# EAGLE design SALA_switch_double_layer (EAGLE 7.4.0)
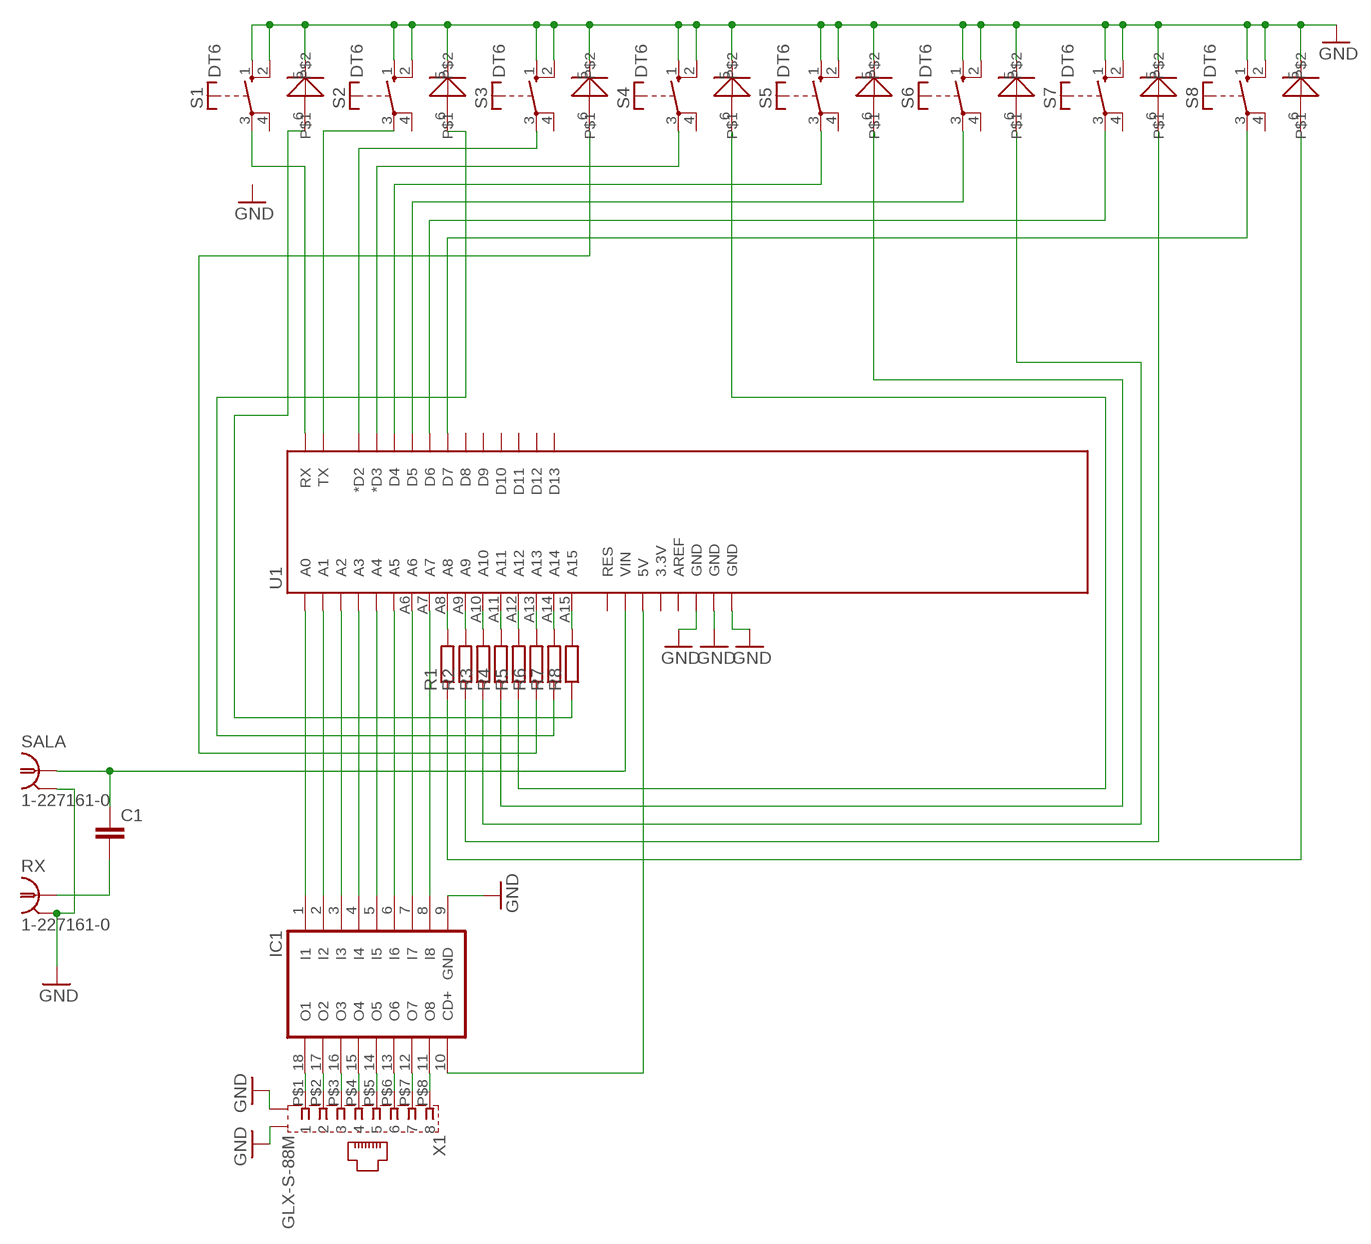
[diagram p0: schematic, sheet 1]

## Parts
C1  C-EU025-024X044  [C025-024X044]
IC1  ULN2803A  [DIL18]
R1  R-EU_R0805  [R0805]
R2  R-EU_R0805  [R0805]
R3  R-EU_R0805  [R0805]
R4  R-EU_R0805  [R0805]
R5  R-EU_R0805  [R0805]
R6  R-EU_R0805  [R0805]
R7  R-EU_R0805  [R0805]
R8  R-EU_R0805  [R0805]
RX  1-227161-0  [AMP_227161]
S1  DT6  [DT6]
S2  DT6  [DT6]
S3  DT6  [DT6]
S4  DT6  [DT6]
S5  DT6  [DT6]
S6  DT6  [DT6]
S7  DT6  [DT6]
S8  DT6  [DT6]
SALA  1-227161-0  [AMP_227161]
U1  ARDUINO_MEGA_SHIELD  [ARDUINO_MEGA_SHIELD]
X1  GLX-S-88M  [GLX-S-88M]

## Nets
GND: IC1.9(GND) RX.2 S1.1(S) S1.2(S) S1.5 S2.1(S) S2.2(S) S2.5 S3.1(S) S3.2(S) S3.5 S4.1(S) S4.2(S) S4.5 S5.1(S) S5.2(S) S5.5 S6.1(S) S6.2(S) S6.5 S7.1(S) S7.2(S) S7.5 S8.1(S) S8.2(S) S8.5 SALA.2 X1.P$9(S1) X1.P$10(S2)
GND@0: U1.GND@0(GND) ; supply symbol labelled GND
GND@1: U1.GND@1(GND) ; supply symbol labelled GND
GND@2: U1.GND@2(GND) ; supply symbol labelled GND
N$1: S1.3(P) U1.RX
N$2: S2.3(P) U1.TX
N$3: S3.3(P) U1.D2(*D2)
N$4: S4.3(P) U1.D3(*D3)
N$5: S5.3(P) U1.D4
N$6: S6.3(P) U1.D5
N$7: S7.3(P) U1.D6
N$8: S8.3(P) U1.D7
N$9: IC1.1(I1) U1.A0
N$10: IC1.2(I2) U1.A1
N$11: IC1.3(I3) U1.A2
N$12: IC1.4(I4) U1.A3
N$13: IC1.5(I5) U1.A4
N$14: IC1.6(I6) U1.A5
N$15: IC1.7(I7) U1.A6
N$16: IC1.8(I8) U1.A7
N$17: R1.2 U1.A8
N$18: R2.2 U1.A9
N$19: R3.2 U1.A10
N$20: R4.2 U1.A11
N$21: R5.2 U1.A12
N$22: R6.2 U1.A13
N$23: R7.2 U1.A14
N$24: R8.2 U1.A15
N$25: R8.1 S1.6
N$26: R7.1 S2.6
N$27: R5.1 S4.6
N$28: R6.1 S3.6
N$29: R3.1 S6.6
N$30: R2.1 S7.6
N$31: C1.1 SALA.1 U1.VIN
N$32: R1.1 S8.6
N$34: R4.1 S5.6
N$35: IC1.10(CD+) U1.5V@0(5V)
N$36: IC1.18(O1) X1.P$1
N$37: IC1.17(O2) X1.P$2
N$38: IC1.16(O3) X1.P$3
N$39: IC1.15(O4) X1.P$4
N$40: IC1.14(O5) X1.P$5
N$41: IC1.13(O6) X1.P$6
N$42: IC1.12(O7) X1.P$7
N$43: IC1.11(O8) X1.P$8
N$44: C1.2 RX.1
Unconnected: S1.4(P) S2.4(P) S3.4(P) S4.4(P) S5.4(P) S6.4(P) S7.4(P) S8.4(P) U1.3.3V U1.AREF U1.D8 U1.D9 U1.D10 U1.D11 U1.D12 U1.D13 U1.RES

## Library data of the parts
C1 = resistor:C-EU: CAPACITOR, European symbol
IC1 = uln-udn:ULN2803A: DRIVER ARRAY
R1-R8 = resistor:R-EU_: RESISTOR, European symbol
RX SALA = con-coax:?227161*: JACK, RIGHT ANGLE, 50 OHM, PCB, BNC; MF: TYCO ELECTRONICS; MPN: 1-227161; OC_FARNELL: unknown; OC_NEWARK: 33B3200
S1-S8 = switch-misc:DT: ITT SWITCH
U1 = RepRapjr:ARDUINO_MEGA_SHIELD
X1 = con-kycon:GLX-S-88M: Mod. Jack, Right Angle, 8 posiotion, 8 contatcs RJ45 Source: GLX-S-88M.pdf; OC_FARNELL: unknown; OC_NEWARK: unknown

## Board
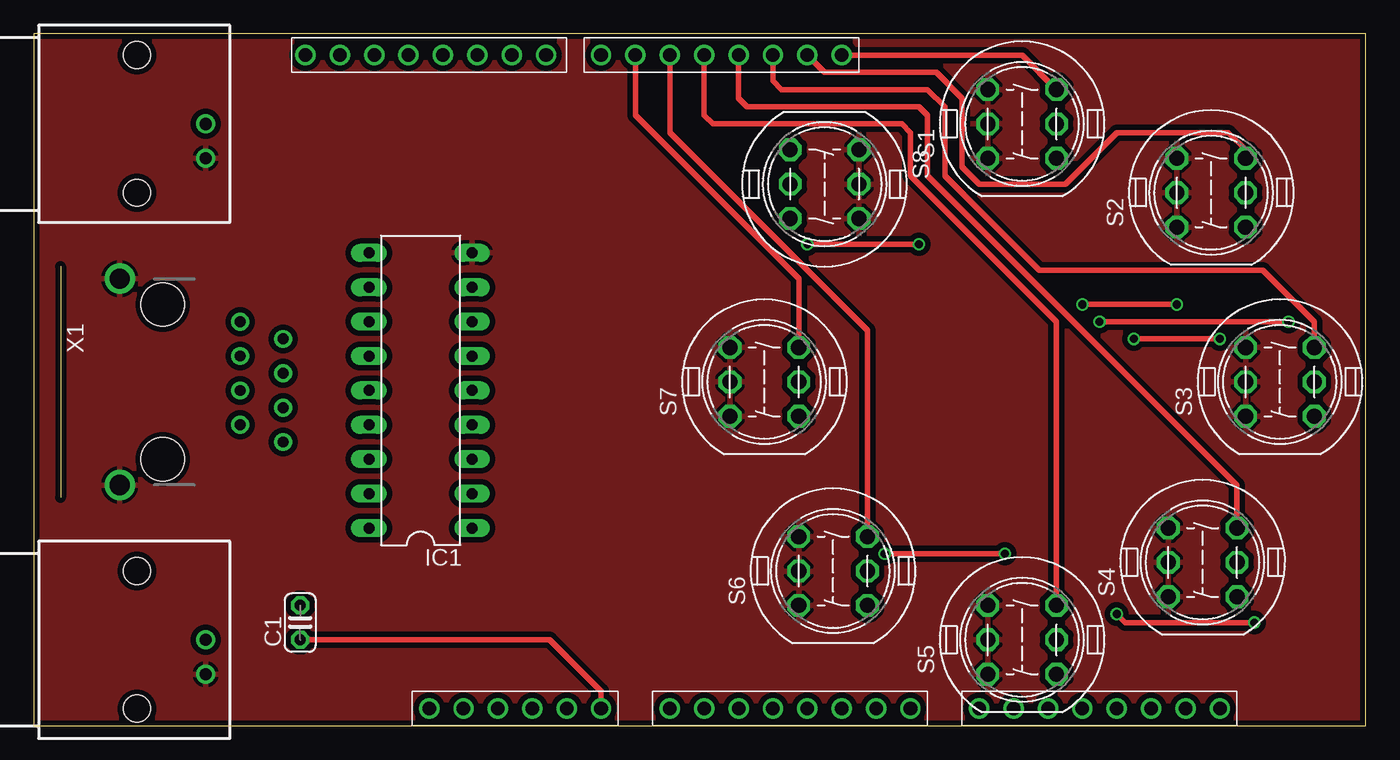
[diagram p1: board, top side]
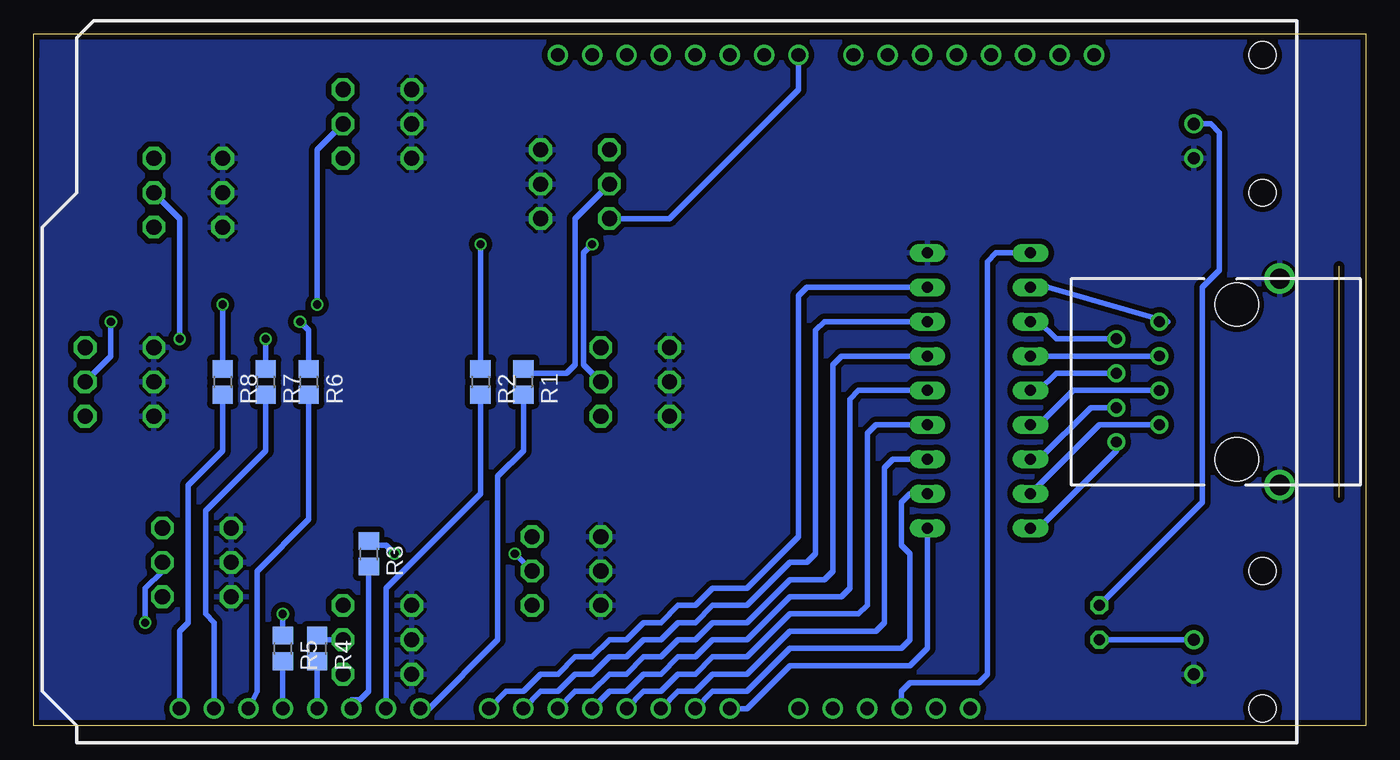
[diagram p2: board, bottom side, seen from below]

Size 98.41 x 51.1 mm. Coordinates in mm from the lower left corner, seen from the top.
Outline: 0,0 98.41,0 98.41,51.1 0,51.1 0,0
Copper layers (1*16): Top 0.035mm / dielectric 1.5mm / Bottom 0.035mm
Design rules "SeeedStudio_2layer_DRU_no_angle_20140221": minimum track width 6mil, minimum drill 12mil, track to track 6mil, track to pad 6mil, pad to pad 6mil, via to via 6mil, smd to smd 0mil, copper to edge 10mil, drill to drill 10mil, minimum pad ring 10mil, minimum via ring 6mil, stop-mask expansion 2mil, vias tented up to drill 100mil, thermal gap 10mil

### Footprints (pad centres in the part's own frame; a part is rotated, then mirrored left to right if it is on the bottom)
C025-024X044 = drill 0.813 octagon: 1 -1.27,0; 2 1.27,0
DIL18 = drill 0.813 long: 1 -10.16,-3.81; 2 -7.62,-3.81; 3 -5.08,-3.81; 4 -2.54,-3.81; 5 0,-3.81; 6 2.54,-3.81; 7 5.08,-3.81; 8 7.62,-3.81; 9 10.16,-3.81; 10 10.16,3.81; 11 7.62,3.81; 12 5.08,3.81; 13 2.54,3.81; 14 0,3.81; 15 -2.54,3.81; 16 -5.08,3.81; 17 -7.62,3.81; 18 -10.16,3.81
R0805 = smd 1.3 x 1.5: 1 -0.95,0; 2 0.95,0
AMP_227161 = drill 0.9 pad 1.27: 1 0,-5.08; 2 -2.54,-5.08 | hole 2: -5.08,0; 5.08,0
DT6 = drill 1.118 octagon: 1 -2.54,2.54; 2 2.54,2.54; 3 2.54,-2.54; 4 -2.54,-2.54; 5 0,2.54; 6 0,-2.54
ARDUINO_MEGA_SHIELD = drill 1 pad 1.422: 3.3V 50.8,26.67; 5V@0 50.8,29.21; A0 50.8,41.91; A1 50.8,44.45; A2 50.8,46.99; A3 50.8,49.53; A4 50.8,52.07; A5 50.8,54.61; A6 50.8,57.15; A7 50.8,59.69; A8 50.8,64.77; A9 50.8,67.31; A10 50.8,69.85; A11 50.8,72.39; A12 50.8,74.93; A13 50.8,77.47; A14 50.8,80.01; A15 50.8,82.55; AREF 2.54,14.986; D2 2.54,49.53; D3 2.54,46.99; D4 2.54,44.45; D5 2.54,41.91; D6 2.54,39.37; D7 2.54,36.83; D8 2.54,32.766; D9 2.54,30.226; D10 2.54,27.686; D11 2.54,25.146; D12 2.54,22.606; D13 2.54,20.066; GND@0 50.8,31.75; GND@1 50.8,34.29; GND@2 2.54,17.526; RES 50.8,24.13; RX 2.54,54.61; TX 2.54,52.07; VIN 50.8,36.83
GLX-S-88M = drill 0.8: P$1 4.445,3.175; P$2 3.175,0; P$3 1.905,3.175; P$4 0.635,0; P$5 -0.635,3.175; P$6 -1.905,0; P$7 -3.175,3.175; P$8 -4.445,0 | drill 1.5: P$9 -7.62,-8.89; P$10 7.62,-8.89 | hole 3.2: -5.715,-5.715; 5.715,-5.715

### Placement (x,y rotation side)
C1  19.69,7.62 90 top
IC1  28.58,24.76 90 top
R1  62.23,25.4 270 bottom
R2  65.41,25.4 270 bottom
R3  73.66,12.7 270 bottom
R4  77.47,5.71 270 bottom
R5  80.01,5.71 270 bottom
R6  78.11,25.4 270 bottom
R7  81.28,25.4 270 bottom
R8  84.45,25.4 270 bottom
RX  7.62,44.45 90 top
S1  73.03,44.45 90 top
S2  87,39.37 90 top
S3  92.08,25.4 90 top
S4  86.36,12.06 90 top
S5  73.03,6.35 90 top
S6  59.06,11.43 90 top
S7  53.98,25.4 90 top
S8  58.42,40.01 270 top
SALA  7.62,6.35 90 top
U1  5.08,52.07 270 top
X1  15.24,25.4 270 top

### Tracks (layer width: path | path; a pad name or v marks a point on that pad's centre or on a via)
GND
  pour Bottom (isolate 0.406): 0,50.8 97.79,50.8 98.42,-0.64 0,0
  pour Top (isolate 0.406): 0,50.8 98.42,50.8 98.42,-0.64 0,0
N$1
  Top 0.406: S1.3 73.03,49.53 U1.RX
N$2
  Top 0.406: S2.3 89.53,42.54 88.27,43.81 80.01,43.81 76.2,40.01 69.85,40.01 68.58,41.27 68.58,46.35 66.67,48.26 58.42,48.26 U1.TX
N$3
  Top 0.406: S3.3 94.61,29.84 90.81,33.65 74.3,33.65 67.31,40.64 67.31,45.72 66.04,46.99 55.25,46.99 54.61,47.62 U1.D2
N$4
  Top 0.406: S4.3 88.9,17.78 66.04,40.64 66.04,45.09 65.41,45.72 52.7,45.72 52.07,46.35 U1.D3
N$5
  Top 0.406: S5.3 75.56,29.84 64.77,40.64 64.77,43.81 64.14,44.45 50.17,44.45 49.53,45.09 U1.D4
N$6
  Top 0.406: S6.3 61.59,29.21 46.99,43.81 U1.D5
N$7
  Top 0.406: S7.3 56.52,33.02 44.45,45.09 U1.D6
N$8
  Bottom 0.406: S8.3 51.44,37.46 41.91,46.99 U1.D7
N$9
  Bottom 0.406: IC1.1 32.39,5.71 33.66,4.45 42.55,4.45 45.72,1.27 U1.A0
N$10
  Bottom 0.406: IC1.2 33.66,17.14 34.29,16.51 34.29,13.33 33.66,12.7 33.66,6.35 34.29,5.71 42.55,5.71 45.72,2.54 48.26,2.54 U1.A1
N$11
  Bottom 0.406: IC1.3 34.93,19.68 35.56,19.05 35.56,7.62 36.2,6.98 42.55,6.98 45.72,3.81 48.26,3.81 49.53,2.54 50.8,2.54 U1.A2
N$12
  Bottom 0.406: IC1.4 36.2,22.22 36.83,21.59 36.83,8.89 37.47,8.25 42.55,8.25 45.72,5.08 48.26,5.08 49.53,3.81 50.8,3.81 52.07,2.54 53.34,2.54 U1.A3
N$13
  Bottom 0.406: IC1.5 37.47,24.76 38.1,24.13 38.1,10.16 38.73,9.52 42.55,9.52 45.72,6.35 48.26,6.35 49.53,5.08 50.8,5.08 52.07,3.81 53.34,3.81 54.61,2.54 55.88,2.54 U1.A4
N$14
  Bottom 0.406: IC1.6 38.73,27.3 39.37,26.67 39.37,11.43 40.01,10.79 42.55,10.79 45.72,7.62 48.26,7.62 49.53,6.35 50.8,6.35 52.07,5.08 53.34,5.08 54.61,3.81 55.88,3.81 57.15,2.54 58.42,2.54 U1.A5
N$15
  Bottom 0.406: IC1.7 40.01,29.84 40.64,29.21 40.64,12.7 41.27,12.06 42.55,12.06 45.72,8.89 48.26,8.89 49.53,7.62 50.8,7.62 52.07,6.35 53.34,6.35 54.61,5.08 55.88,5.08 57.15,3.81 58.42,3.81 59.69,2.54 60.96,2.54 U1.A6
N$16
  Bottom 0.406: IC1.8 41.27,32.38 41.91,31.75 41.91,13.97 45.72,10.16 48.26,10.16 49.53,8.89 50.8,8.89 52.07,7.62 53.34,7.62 54.61,6.35 55.88,6.35 57.15,5.08 58.42,5.08 59.69,3.81 60.96,3.81 62.23,2.54 63.5,2.54 U1.A7
N$17
  Bottom 0.406: R1.2 62.23,20.32 64.14,18.41 64.14,6.35 69.22,1.27 U1.A8
N$18
  Bottom 0.406: R2.2 65.41,17.14 72.39,10.16 U1.A9
N$19
  Bottom 0.406: R3.2 73.66,2.54 74.3,1.9 74.93,1.9 U1.A10
N$20
  Bottom 0.406: U1.A11 R4.2
N$21
  Bottom 0.406: U1.A12 R5.2
N$22
  Bottom 0.406: R6.2 78.11,15.24 81.92,11.43 81.92,2.54 U1.A13
N$23
  Bottom 0.406: R7.2 81.28,20.32 85.73,15.88 85.73,8.25 85.09,7.62 U1.A14
N$24
  Bottom 0.406: R8.2 84.45,20.32 87,17.78 87,7.62 87.63,6.98 U1.A15
N$25  (via drill 0.6)
  Top 0.406: v84.45,31.12 v77.47,31.12
  Bottom 0.406: S1.6 77.47,42.54 v77.47,31.12 | R8.1 v84.45,31.12
N$26  (via drill 0.6)
  Top 0.406: v81.28,28.57 v87.63,28.57
  Bottom 0.406: S2.6 87.63,37.46 v87.63,28.57 | R7.1 v81.28,28.57
N$27  (via drill 0.6)
  Top 0.406: v90.17,7.62 80.64,7.62 v80.01,8.25
  Bottom 0.406: S4.6 88.9,11.43 90.17,10.16 v90.17,7.62 | R5.1 v80.01,8.25
N$28  (via drill 0.6)
  Top 0.406: v78.74,29.84 v92.71,29.84
  Bottom 0.406: S3.6 92.71,27.3 v92.71,29.84 | v78.74,29.84 78.11,29.21 R6.1
N$29  (via drill 0.6)
  Top 0.406: v71.75,12.7 v62.86,12.7
  Bottom 0.406: v62.86,12.7 S6.6 | v71.75,12.7 72.39,13.33 73.66,13.33 R3.1
N$30  (via drill 0.6)
  Top 0.406: v65.41,35.56 v57.15,35.56
  Bottom 0.406: S7.6 57.78,26.67 57.78,34.92 v57.15,35.56 | R2.1 v65.41,35.56
N$31
  Top 0.406: U1.VIN 41.91,2.54 38.1,6.35 C1.1
  Bottom 0.406: C1.1 SALA.1
N$32
  Bottom 0.406: S8.6 58.42,37.46 58.42,26.67 59.06,26.03 62.23,26.03 R1.1
N$34
  Bottom 0.406: S5.6 77.79,6.35 R4.1
N$35
  Bottom 0.406: IC1.10 27.3,34.92 27.94,34.29 27.94,3.81 28.58,3.17 33.66,3.17 34.29,2.54 U1.5V@0
N$36
  Bottom 0.406: IC1.18 24.13,14.6 18.41,20.32 X1.P$1
N$37
  Bottom 0.406: IC1.17 19.69,22.22 X1.P$2
N$38
  Bottom 0.406: IC1.16 24.13,19.68 20.32,23.49 X1.P$3
N$39
  Bottom 0.406: IC1.15 24.13,22.22 21.59,24.76 X1.P$4
N$40
  Bottom 0.406: IC1.14 24.13,24.76 22.86,26.03 X1.P$5
N$41
  Bottom 0.406: IC1.13 X1.P$6
N$42
  Bottom 0.406: IC1.12 24.13,29.84 22.86,28.57 X1.P$7
N$43
  Bottom 0.406: X1.P$8 14.61,29.84 23.5,32.38 IC1.11
N$44
  Bottom 0.406: RX.1 11.43,44.45 10.8,43.81 10.8,33.65 12.07,32.38 12.07,16.51 C1.2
